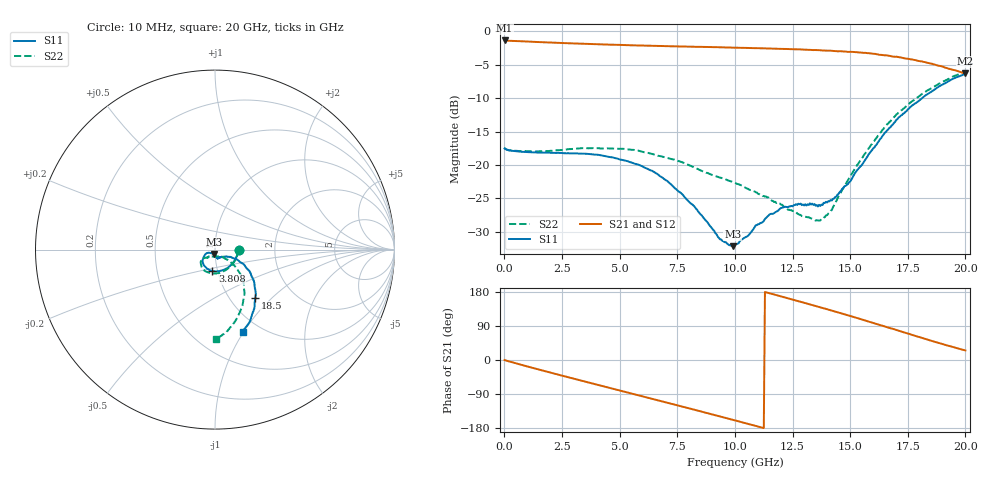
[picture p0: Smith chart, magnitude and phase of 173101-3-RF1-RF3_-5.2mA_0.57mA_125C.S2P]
!  2-Port S-parameters saved by WinCal
! VAR MeasName=S-Parameters (CALIBRATED_DATA) read from VNA (N5242A)
! VAR MeasDate=2017-7-20 10:52:37
! VAR NAME=173101-3-RF1-RF3_-5.2mA_0.57mA_125C
! VAR FILENAME=173101-3-RF1-RF3_-5.2mA_0.57mA_125C.S2P
! VAR DATE=2017-7-20 10:52:37
! VAR PHYS_PORTS=1,2
# Hz S DB R 50
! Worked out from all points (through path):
!   401 points, 10 MHz to 20 GHz, reference 50 ohm
!   highest |S21| = -1.37 dB at 10 MHz (marker M1); lowest = -6.3 dB at 20 GHz (marker M2)
!   group delay of S21, straight-line fit = 46 ps
!   lowest |S11| = -32.1 dB at 9.905 GHz (marker M3), VSWR 1.05, Z = 49.2 - j2.33 ohm
!   |S11| at or under -10 dB: start of sweep to 18.11 GHz
!   |S22| runs from -28.3 to -6.0 dB; largest |S21 - S12| = 0.0065
!   S11 on the Smith chart (normalised r, x): 10 MHz: 1.31, -0.01; 3.808 GHz: 0.94, -0.23; 18.5 GHz: 1.30, -0.80; 20 GHz: 0.83, -0.99
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1e7  -17.53 -1.0  -1.37 -0.2  -1.37 -0.2  -17.48 -1.0
1.559225e9  -18.14 -45.6  -1.62 -26.2  -1.62 -26.2  -17.95 -44.9
2.50875e9  -18.21 -69.2  -1.75 -41.4  -1.76 -41.4  -17.75 -67.6
3.358325e9  -18.30 -88.4  -1.87 -54.8  -1.87 -54.8  -17.47 -84.8
3.8081e9  -18.41 -97.0  -1.91 -61.8  -1.92 -61.8  -17.48 -92.6
5.2074e9  -19.30 -123.1  -2.07 -83.7  -2.08 -83.6  -17.58 -114.7
6.70665e9  -21.54 -142.4  -2.19 -107.1  -2.18 -107.0  -18.64 -131.0
8.4058e9  -26.94 -156.0  -2.32 -133.7  -2.34 -133.7  -20.61 -142.7
9.355325e9  -31.11 -133.5  -2.40 -149.0  -2.40 -149.0  -21.89 -142.8
9.90505e9  -32.14 -106.8  -2.44 -157.8  -2.45 -157.8  -22.55 -141.5
1.0005e10  -31.96 -103.1  -2.45 -159.4  -2.46 -159.4  -22.67 -141.2
1.105448e10  -28.84 -80.2  -2.53 -176.4  -2.54 -176.4  -24.36 -133.5
1.205398e10  -26.38 -78.1  -2.63 167.1  -2.64 167.1  -25.95 -127.3
1.335332e10  -25.77 -67.7  -2.79 145.1  -2.77 145.1  -28.04 -97.8
1.38031e10  -25.99 -58.3  -2.88 137.2  -2.87 137.2  -28.11 -77.1
1.410295e10  -25.44 -49.2  -2.89 132.1  -2.92 132.0  -27.12 -58.8
1.44028e10  -24.73 -43.8  -2.97 126.8  -2.99 126.9  -25.38 -49.5
1.555222e10  -19.77 -24.8  -3.21 106.1  -3.23 105.9  -18.80 -38.9
1.670165e10  -14.46 -28.1  -3.66 84.7  -3.72 84.4  -13.58 -45.5
1.76012e10  -11.35 -37.8  -4.16 68.2  -4.16 68.1  -10.68 -55.8
1.850075e10  -9.10 -50.2  -4.82 51.1  -4.88 51.1  -8.56 -68.2
2e10  -6.33 -71.4  -6.30 25.3  -6.36 25.8  -6.04 -89.1
